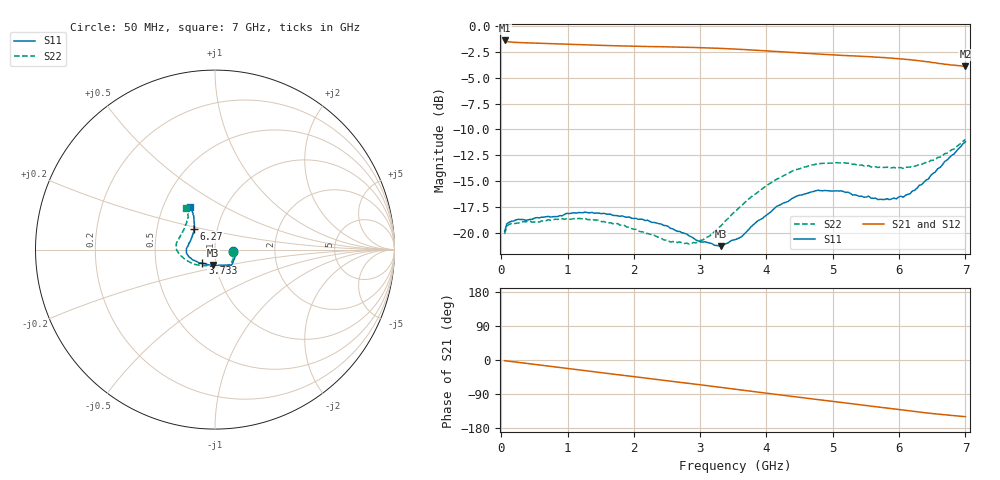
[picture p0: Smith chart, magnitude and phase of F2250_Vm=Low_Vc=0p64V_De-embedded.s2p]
! Integrated Device Technology
! Corporate Headquarters
! 6024 Silver Creek Valley Road
! San Jose, CA 95138  USA
! Phone:  1-408-284-8200
! Toll Free:  1-800-223-1366
! Webpage:  http://www.idt.com/
! Timing and RF Division
! 515 Groton Road, Suite 102
! Westford, MA 01886-6024
! Device:  F2250
! Description: Voltage Variable RF Attenuator
! Frequency:  50.0 -  6000.00 MHz
! Package:  3x3 mm Thin QFN Plastic Package: 16 pin
! Ports:  2 RF, 3 DC
!  Pin  1  = GND
!  Pin  2  = NC
!  Pin  3  = RF1  = Port 1
!  Pin  4  = NC
!  Pin  5  = GND
!  Pin  6  = GND
!  Pin  7  = GND
!  Pin  8  = GND
!  Pin  9  = NC
!  Pin 10  = RF2  = Port 2
!  Pin 11  = NC
!  Pin 12  = GND
!  Pin 13  = GND
!  Pin 14  = VCNTRL
!  Pin 15  = VDD
!  Pin 16  = VMODE
! Vcntrl:  0.640 Volts
! Vmode:  +0.000 Volts
! Vdd:  +3.30  Volts
! Current:  1.142 mA
! Data:  The device was measured on a the F2250 evaluation board which has
!  individual transmission lines to the RF pins.  Data was collected
!  using a calibrated network analyzer.  The evaluation board was
!  de-embedded using a TRL calibration technique.
!  The reference plane is the edge of the package pin.
! Misc:  SN 10
!  Action Tracker AT0258
! Date Measured:  2014-11-26
! Date:  2015-10-15  MJV
! Note:
!  Integrated Device Technology supplies this data as a sample of measured
!  data at the package pin for this product.  Your particular data for this
!  product may vary.
!  Data was taken at 25 degrees C.
!  Integrated Device Technology reserves the right to change this data at anytime.
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# GHz S dB R 50
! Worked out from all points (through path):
!   201 points, 50 MHz to 7 GHz, reference 50 ohm
!   highest |S21| = -1.40 dB at 50 MHz (marker M1); lowest = -3.9 dB at 7 GHz (marker M2)
!   group delay of S21, straight-line fit = 60 ps
!   lowest |S11| = -21.3 dB at 3.317 GHz (marker M3), VSWR 1.19, Z = 48.1 - j8.26 ohm
!   |S11| at or under -10 dB: start of sweep to end of sweep
!   |S22| runs from -21.1 to -11.0 dB; largest |S21 - S12| = 0.0007
!   S11 on the Smith chart (normalised r, x): 50 MHz: 1.22, -0.02; 3.733 GHz: 0.86, -0.13; 6.27 GHz: 0.77, +0.18; 7 GHz: 0.69, +0.35
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0.05  -19.87 -5.2  -1.40 -1.8  -1.40 -1.8  -20.12 -6.6
0.08475  -19.12 -5.5  -1.51 -2.5  -1.50 -2.5  -19.35 -6.4
0.15425  -18.88 -7.5  -1.56 -4.0  -1.56 -4.0  -19.12 -8.2
0.745  -18.48 -27.8  -1.71 -17.0  -1.71 -17.0  -18.79 -33.0
1.2315  -18.06 -41.2  -1.82 -27.5  -1.82 -27.5  -18.66 -50.7
1.75275  -18.35 -48.2  -1.92 -38.5  -1.92 -38.5  -19.10 -61.3
2.37825  -19.12 -51.6  -2.01 -51.8  -2.01 -51.8  -20.45 -71.9
2.552  -19.57 -54.6  -2.03 -55.6  -2.02 -55.6  -20.90 -77.8
2.93425  -20.69 -68.5  -2.09 -64.0  -2.09 -64.0  -20.97 -98.5
3.14275  -20.98 -82.8  -2.13 -68.6  -2.13 -68.6  -20.31 -113.8
3.3165  -21.30 -98.1  -2.17 -72.5  -2.17 -72.5  -19.31 -125.0
3.525  -20.67 -115.8  -2.24 -77.1  -2.24 -77.1  -17.97 -137.1
3.7335  -19.67 -132.6  -2.31 -81.8  -2.31 -81.8  -16.73 -147.0
4.1505  -17.46 -153.6  -2.48 -91.0  -2.47 -91.0  -14.84 -164.6
4.46325  -16.42 -164.5  -2.60 -97.8  -2.60 -97.8  -13.87 -173.7
4.7065  -16.01 -171.5  -2.69 -103.0  -2.69 -103.0  -13.44 -179.5
5.1235  -15.94 178.4  -2.84 -112.0  -2.84 -112.0  -13.24 171.3
5.85325  -16.80 153.3  -3.10 -127.5  -3.10 -127.6  -13.74 154.3
6.06175  -16.56 144.7  -3.20 -132.1  -3.20 -132.1  -13.78 148.2
6.27025  -15.69 135.4  -3.34 -136.6  -3.34 -136.6  -13.50 141.6
6.61775  -13.68 124.0  -3.64 -143.3  -3.64 -143.3  -12.70 129.9
7  -11.20 119.7  -3.90 -149.5  -3.91 -149.5  -10.99 125.4
